(* Logix 5000 AddOnInstructionDefinition export MTRQ_Yaskawa; software revision 17.00 *)

TYPE Yaskawa_EIP_Servo :   // Yaskawa SigmaLogic Axis Structure v2.4.0
STRUCT
   O : Yaskawa_OUT_to_Servo;
   I : Yaskawa_IN_from_Servo;
   AOI_SB : Yaskawa_AOI_Status_Bits;
END_STRUCT
END_TYPE

TYPE Yaskawa_OUT_to_Servo :   // Structure of data sent out to the Yaskawa SigmaLogic controller v2.4.0
STRUCT
   b00_ServoOn : BOOL;   // Servo On
   b01_Stop : BOOL;   // Stops All Current Motion in Progress
   b02_Home : BOOL;   // Start Homing Process
   b03_MoveStart1 : BOOL;   // Start Current Motion
   b06_SuperImpose : BOOL;
   b07_ServoAlarmReset : BOOL;   // Servo Alarm Reset
   b08_ControllerAlarmReset : BOOL;   // SigmaLogic Alarm Reset
   b09_MoveStart2 : BOOL;   // Start Second Motion (Blended Move)
   b10_MoveAbort : BOOL;   // Abort Current Move
   b11_MovePause : BOOL;   // Pause Current Move
   b12_SeqPause : BOOL;   // Indexing Sequence Pause
   b13_SeqResume : BOOL;   // Indexing Sequence Resume
   b14_SeqCancel : BOOL;   // Indexing Sequence Cancel
   b15_AbsEncoderReset : BOOL;   // Absolute Encoder Reset
   b16_SeqStart : BOOL;   // Start Indexing Sequence
   b17_SeqEditSpeed : BOOL;   // Enter Edit Speed
   b18_SeqEditDistance : BOOL;   // Enter Distance Edit
   b19_PLSEnable : BOOL;   // Enable PLS execution
   b20_PLSActivateOutput1 : BOOL;   // Activate PLS output1 switch logic
   b21_PLSActivateOutput2 : BOOL;   // Activate PLS output2 switch logic
   b22_PLSActivateOutput3 : BOOL;   // Activate PLS output3 switch logic
   b23_PLSActivateOutput4 : BOOL;   // Activate PLS output4 switch logic
   b24_SetClock : BOOL;   // Set the remote controller clock with data provided by the PLC
   RebootController : BOOL;
   UseExternalEncoder : BOOL;   // Use External Encoder when executing MAHSP_Yaskawa
   b32_HeatbeatAnswer : BOOL;   // Heartbeat Answer
   BrakeBypassRequest : BOOL;
   SetFwdTorqueLimit : BOOL;
   SetRevTorqueLimit : BOOL;
   TorqueLimit : DINT;
   TorqueRamp : DINT;
   HomeMethod : INT;
   HomeSpeed : DINT;
   HomeAccDec : DINT;   // Home Move Acceleration/Deceleration Rate
   HomeBackOffDistance : DINT;
   HomeCreepSpeed : DINT;
   HomeCreepDistanceLimit : DINT;
   HomeCreepTimeLimit : DINT;
   HomeOffsetDistance : DINT;
   HomeOffsetSpeed : DINT;
   HomePostion : DINT;
   HomeTorque : DINT;
   HomeInputNo : DINT;
   HomeApproachTimeLimit : DINT;
   HomeApproachDistLimit : DINT;
   HomeDirection : INT;
   HomeSwitchMode : INT;
   MoveType : INT;
   MoveDirection : INT;
   MoveAccel1 : DINT;
   MoveAccel2 : DINT;
   MoveDecel1 : DINT;
   MoveDecel2 : DINT;
   MoveSpeed1 : DINT;
   MoveSpeed2 : DINT;
   MoveDistance1 : DINT;
   MoveDistance2 : DINT;
   MovePosition1 : DINT;
   MovePosition2 : DINT;
   RegistrationDistance : DINT;
   GearNumerator : DINT;
   GearDenominator : DINT;
   SuperImposeDistance : DINT;
   Resolution : INT;
   RegistrationDirection : INT;
   TuningLevel : INT;
   SequenceStep : INT;   // Staring Sequence Step Number
   SequenceEditStep : INT;   // Sequence Step Number to Edit
   FlagCommandBits1 : DINT;   // Flag Commands. 1..64 are General Flags, Bits 0..31 correspond to Flag 1..32
   FlagCommandBits2 : DINT;   // Flag Commands cont. 1..64 are General Flags, Bits 0..31 correspond to Flag 33..64
   DigitalOutCommandBits : DINT;   // Digital Output commands. Bits 0-7 correspond to CN13 Digital Outputs 0-7, used as Flag 73-80. Bits 8-10 correspond to CN1 Digital Outputs 0-2 used as Flag 88-90"
   SequenceEditSpeed : DINT;
   SequenceEditDistance : DINT;
   FeedRateOverride : INT;
   HSI_Enable : BOOL;
   HSI_MoveMode : BOOL;   // 0=Relative; 1=Moves per Cycle
   HSI_CalcMethod : BOOL;   // 0=Accel/Decel; 1=Time
   HSI_MoveDirection : BOOL;   // 0 = Negative; 1 = Positive
   HSI_TriggerFlag : INT;
   HSI_MovingFlag : INT;
   HSI_DwellingFlag : INT;
   HSI_DoneFlag : INT;
   HSI_MoveType : INT;   // 0=Single; 1=Repeat; 2=Repeat "x" times
   HSI_RepeatNumber : INT;
   HSI_Distance : DINT;
   HSI_Speed : DINT;
   HSI_Accel : DINT;
   HSI_MoveTime : DINT;
   HSI_DwellTime : DINT;
   PLS_OutputFlag1 : INT;
   PLS_OutputFlag2 : INT;
   PLS_OutputFlag3 : INT;
   PLS_OutputFlag4 : INT;
   PLS_OnPosition1 : DINT;
   PLS_OffPosition1 : DINT;
   PLS_OnPosition2 : DINT;
   PLS_OffPosition2 : DINT;
   PLS_OnPosition3 : DINT;
   PLS_OffPosition3 : DINT;
   PLS_OnPosition4 : DINT;
   PLS_OffPosition4 : DINT;
   PLS_OnCompensation1 : INT;
   PLS_OffCompensation1 : INT;
   PLS_OnCompensation2 : INT;
   PLS_OffCompensation2 : INT;
   PLS_OnCompensation3 : INT;
   PLS_OffCompensation3 : INT;
   PLS_OnCompensation4 : INT;
   PLS_OffCompensation4 : INT;
   RTC_Year : INT;
   RTC_Month : INT;
   RTC_Day : INT;
   RTC_Hour : INT;
   RTC_Min : INT;
   RTC_Sec : INT;
   StopDecel : DINT;
   AnalogOutput : INT;   // CN13, AO_01 [mV]
END_STRUCT
END_TYPE

TYPE Yaskawa_AOI_Status_Bits :   // Internal bits used to interlock Yaskawa AOI execution. v2.4.0
STRUCT
   MAM : BOOL;   // Move AOI Active
   MAJ : BOOL;   // Jog AOI Active
   MAB : BOOL;   // Blending AOI Active
   MAG : BOOL;   // Gearing AOI Active
   MAHSP : BOOL;   // Home SetPoint AOI Active
   MAH : BOOL;   // Homing AOI Active
   MSQE : BOOL;   // Sequence Edit AOI Active
   MSQR : BOOL;   // Sequence Run AOI Active
   MHSI : BOOL;   // High Speed Index AOI Active
   MSO : BOOL;   // Servo On
   MSF : BOOL;   // Servo Off
   MAFR : BOOL;   // Fault Reset
   MAS : BOOL;   // Servo Abort
   MTRQ : BOOL;   // Torque Mode Active
   MPLS : BOOL;   // PLS Active
   MCLK : BOOL;   // SetClock Active
   MSTL : BOOL;   // Set Torque Limit Active
   AOI_Permissive : BOOL;   // Permissive to Execute an AOI
END_STRUCT
END_TYPE

TYPE Yaskawa_IN_from_Servo :   // Structure of data coming from the Yaskawa SigmaLogic controller. v2.4.0
STRUCT
   AlarmText : STRING;   // ServoPack Alarm Code plus Text Description
   b00_Heartbeat : BOOL;
   b01_Alarm : BOOL;   // ServoPack Alarm
   b02_Warning : BOOL;   // ServoPack Warning
   b03_Ready : BOOL;   // ServoPack Ready
   b04_Enabled : BOOL;   // ServoPack Enabled ("Servo On")
   b05_StopComplete : BOOL;
   b06_HomeComplete : BOOL;
   b07_HomeBusy : BOOL;
   b08_HomeActive : BOOL;
   b09_HomeAborted : BOOL;
   b10_HomeError : BOOL;
   b11_MoveAbsComplete : BOOL;
   b12_MoveAbsBusy : BOOL;
   b13_MoveAbsActive : BOOL;
   b14_MoveAbsAborted : BOOL;
   b15_MoveAbsError : BOOL;
   b16_MoveRelComplete : BOOL;
   b17_MoveRelBusy : BOOL;
   b18_MoveRelActive : BOOL;
   b19_MoveRelAborted : BOOL;
   b20_MoveRelError : BOOL;
   b21_JogAtSpeed : BOOL;
   b22_JogBusy : BOOL;
   b23_JogActive : BOOL;
   b24_JogAborted : BOOL;
   b25_JogError : BOOL;
   b26_GearInSync : BOOL;
   b27_GearBusy : BOOL;
   b28_GearActive : BOOL;
   b29_GearAborted : BOOL;
   b30_GearError : BOOL;
   b32_MoveSuperComplete : BOOL;
   b33_MoveSuperBusy : BOOL;
   b34_MoveSuperActive : BOOL;
   b35_MoveSuperAborted : BOOL;
   b36_MoveSuperError : BOOL;
   b37_PowerCycleRequired : BOOL;
   b38_MoveBlend1Complete : BOOL;
   b39_MoveBlend1Busy : BOOL;
   b40_MoveBlend1Active : BOOL;
   b41_MoveBlend1Abort : BOOL;
   b42_MoveBlend1Error : BOOL;
   b43_MoveBlend2Complete : BOOL;
   b44_MoveBlend2Busy : BOOL;
   b45_MoveBlend2Active : BOOL;
   b46_MoveBlend2Abort : BOOL;
   b47_MoveBlend2Error : BOOL;
   b48_RegComplete : BOOL;
   b49_RegBusy : BOOL;
   b50_RegActive : BOOL;
   b51_RegAborted : BOOL;
   b52_RegError : BOOL;
   b53_ResetAbsEncoderActive : BOOL;
   b54_ResetAbsEncoderBusy : BOOL;
   b55_ResetAbsEncoderDone : BOOL;
   b56_ResetAbsEncoderError : BOOL;
   b57_SeqRunning : BOOL;
   b58_RegSensorNotReached : BOOL;
   b59_SeqEditError : BOOL;
   b60_SeqEditDone : BOOL;
   b61_TorqueAtTorque : BOOL;
   b62_TorqueBusy : BOOL;
   b63_TorqueActive : BOOL;
   b64_TorqueAborted : BOOL;
   b65_TorqueError : BOOL;
   b66_ControllerAlarm : BOOL;
   b67_ApplicationError : BOOL;
   b68_AxisAtStandStill : BOOL;
   b69_TestModeActive : BOOL;
   b70_ServoParamsOK : BOOL;
   b71_SetFwdTorqueLimitDone : BOOL;
   b72_SetRevTorqueLimitDone : BOOL;
   Position : DINT;
   Speed : DINT;
   Torque : DINT;
   HomeErrorID : INT;
   MoveAbsErrorID : INT;
   MoveRelErrorID : INT;
   JogErrorID : INT;
   GearErrorID : INT;
   MoveSuperErrorID : INT;
   ServoAlarmID : INT;
   ServoWarningID : INT;
   ControllerAlarmID : DINT;
   AxisGenAlarmID : DINT;
   MoveBlend1ErrorID : INT;
   MoveBlend2ErrorID : INT;
   ResetAbsEncoderErrorID : INT;
   FunctionBlockErrorID : INT;
   TorqueErrorID : INT;
   RegErrorID : INT;
   SeqCurrentStep : INT;
   FlagStatusBit1 : DINT;   // Flag Status. 1..64 are General Flags, Bits 0..31 correspond to Flag 1..32
   FlagStatusBit2 : DINT;   // Flag Status cont. 1..64 are General Flags, Bits 0..31 correspond to Flag 33..64
   IOStatusBits : DINT;   // Digital IO Status. Bits 0-7, CN13 Inputs 0-7, Used as Flag 65-72. Bits 8-15, CN13 Outputs 0-7, Used as Flag 73-80. Bits 16-22, CN1 Inputs 0-6, Used as Flag 81-87. Bits 23-25, CN1 Outputs 0-4, Used as Flag 88-92.
   HSI_Moving : BOOL;
   HSI_Dwelling : BOOL;
   HSI_Done : BOOL;
   HSI_Busy : BOOL;
   HSI_Error : BOOL;
   HSI_ErrorCode : INT;
   PLS_Running : BOOL;
   PLS_SwitchStatus1 : BOOL;
   PLS_SwitchStatus2 : BOOL;
   PLS_SwitchStatus3 : BOOL;
   PLS_SwitchStatus4 : BOOL;
   PLS_Busy : BOOL;
   PLS_Error : BOOL;
   PLS_ErrorCode : INT;
   SetClock_Done : BOOL;
   SetClock_Busy : BOOL;
   SetClock_Error : BOOL;
   SetClock_ErrorID : INT;
   SoftwareVersion : DINT;
   FirmwareVersion : DINT;
   CommandedPos : DINT;
   CommandedPosNonCyc : DINT;
   CommandedSpeed : DINT;
   Clock_Year : INT;
   Clock_Month : INT;
   Clock_Day : INT;
   Clock_Hour : INT;
   Clock_Minute : INT;
   Clock_Second : INT;
   AnalogInput : REAL;   // CN13, AI_01 [v]
   BrakeBypassActive : BOOL;
   ForwardTorqueLimit : DINT;
   ReverseTorqueLimit : DINT;
END_STRUCT
END_TYPE

ADD_ON_INSTRUCTION MTRQ_Yaskawa   (* revision 2.4 0, vendor Yaskawa America, Inc., ExecuteEnableInFalse *)
// Motion Axis Torque Control
// Revision note:
// 2.4.0: No functional change
// 2.3.1: Moved unlatch of AOI_ON_LOCAL to bottom of EnableInFalse routine so that outputs will be on for at least 1 scan if one-shot on EN is used.
// 2.3.0: No functional change
// 2.0.0: Improved output operation and error code reporting. Improved interlocking with embedded code.
// 1.2.0: Set the IP output to non-latch so that it can show correct status if torque command is changed.
// 1.1.0: Initial Release 9/10/2014
// Help:
// This AOI moves a servo axis indefinitely at a commanded maximum torque with an overall speed limit. The polarity of the torque determines the direction of motion. The motor speed will vary depending on the amount of resistance to motion present in the system. When the maximum torque value is reached, the IP output will signal 'In-Torque'.
VAR_IN_OUT
   Axis : Yaskawa_EIP_Servo; {required}
END_VAR
VAR_INPUT
   Torque_Limit : REAL := 50.0; {required}   // Torque Limit [%] during motion. Positive value is forward direction, Negative value is reverse direction.
   Torque_Ramp : REAL := 100.0; {required}   // Torque Ramp Rate [%/sec]
   Speed_Limit : REAL; {required}   // Maximum Absolute Speed to move the axis in [unit/s]
   Accel_Rate : REAL; {required}   // Acceleration rate of the axis in [unit/s/s]
   Decel_Rate : REAL; {required}   // Deceleration rate of the axis in [unit/s/s]
END_VAR
VAR_OUTPUT
   EN : BOOL; {visible}   // The AOI is Active
   IP : BOOL; {visible}   // The axis is holding "At Torque"
   ER : BOOL; {visible}   // An error has occurred with the Torque Control Motion
   FLT_RDY : BOOL; {visible}   // The Servo is Not Ready
   FLT_BSY : BOOL; {visible}   // There is another AOI Active for this Axis
   ErrorCode : INT; {visible}   // Torque Control ErrorID returned from the SigmaLogic axis
END_VAR
VAR
   AOI_ON_LOCAL : BOOL;
   Move_TORQUE : BOOL;
   ScaleFactor : DINT;
   stopping : BOOL;
   Finished : BOOL;   // Function is Finished
END_VAR

ROUTINE EnableInFalse   (* ladder *)
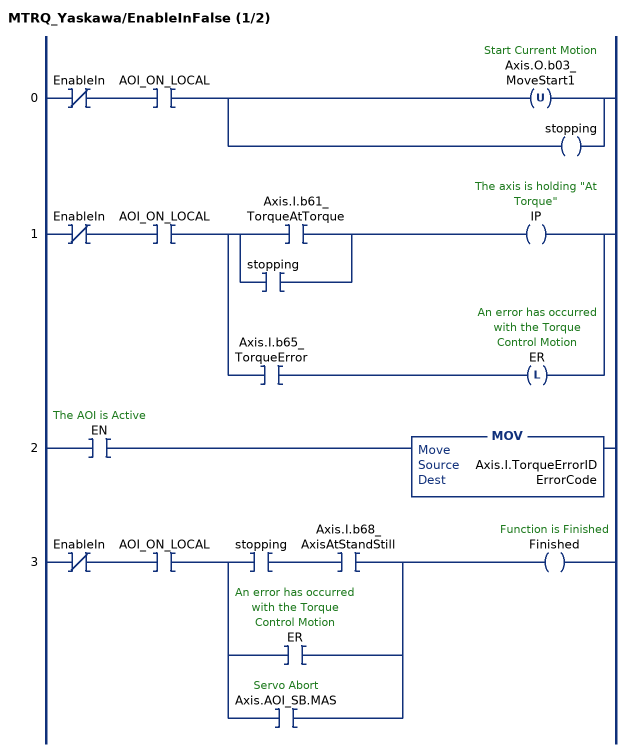
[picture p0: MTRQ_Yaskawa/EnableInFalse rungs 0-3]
   0: XIO(EnableIn)XIC(AOI_ON_LOCAL)[OTU(Axis.O.b03_MoveStart1) ,OTE(stopping) ];
   1: XIO(EnableIn)XIC(AOI_ON_LOCAL)[[XIC(Axis.I.b61_TorqueAtTorque) ,XIC(stopping) ] OTE(IP) ,XIC(Axis.I.b65_TorqueError) OTL(ER) ];
   2: XIC(EN)MOV(Axis.I.TorqueErrorID,ErrorCode);
   3: XIO(EnableIn)XIC(AOI_ON_LOCAL)[XIC(stopping) XIC(Axis.I.b68_AxisAtStandStill) ,XIC(ER) ,XIC(Axis.AOI_SB.MAS) ]OTE(Finished);
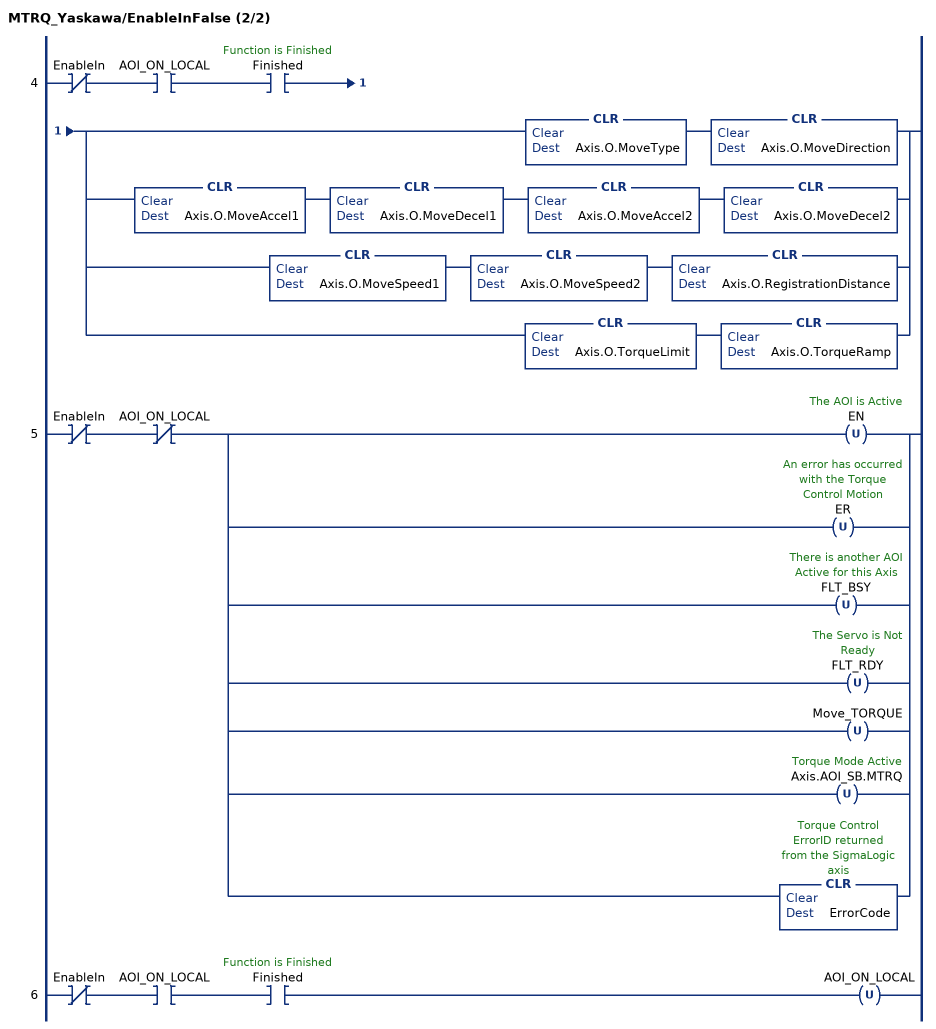
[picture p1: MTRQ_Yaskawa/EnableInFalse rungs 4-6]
   4: XIO(EnableIn)XIC(AOI_ON_LOCAL)XIC(Finished)[CLR(Axis.O.MoveType) CLR(Axis.O.MoveDirection) ,CLR(Axis.O.MoveAccel1) CLR(Axis.O.MoveDecel1) CLR(Axis.O.MoveAccel2) CLR(Axis.O.MoveDecel2) ,CLR(Axis.O.MoveSpeed1) CLR(Axis.O.MoveSpeed2) CLR(Axis.O.RegistrationDistance) ,CLR(Axis.O.TorqueLimit) CLR(Axis.O.TorqueRamp) ];
   5: XIO(EnableIn)XIO(AOI_ON_LOCAL)[OTU(EN) ,OTU(ER) ,OTU(FLT_BSY) ,OTU(FLT_RDY) ,OTU(Move_TORQUE) ,OTU(Axis.AOI_SB.MTRQ) ,CLR(ErrorCode) ];
   6: XIO(EnableIn)XIC(AOI_ON_LOCAL)XIC(Finished)OTU(AOI_ON_LOCAL);
END_ROUTINE

ROUTINE Logic   (* ladder *)
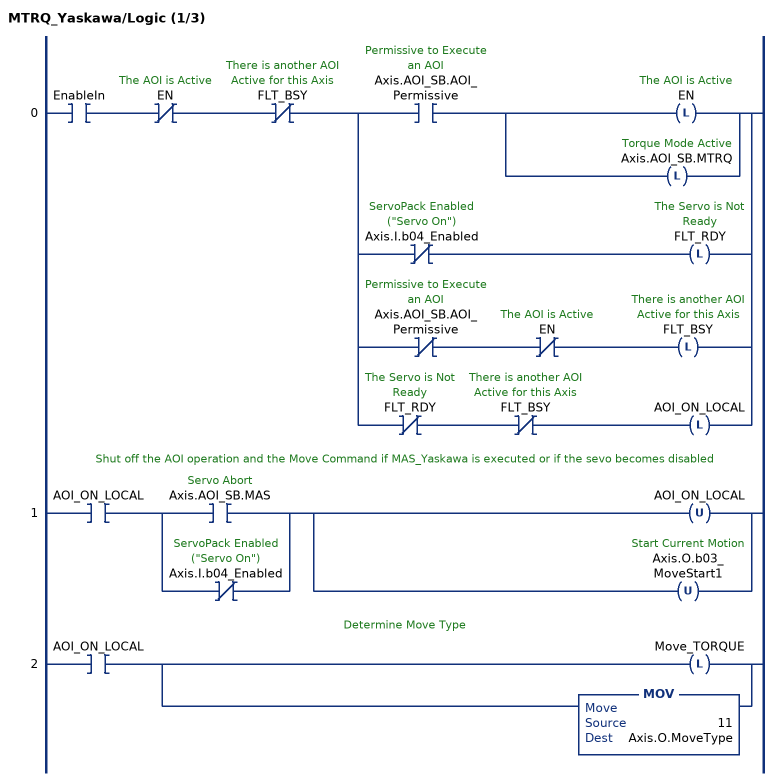
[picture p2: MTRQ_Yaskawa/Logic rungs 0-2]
   0: XIC(EnableIn)XIO(EN)XIO(FLT_BSY)[XIC(Axis.AOI_SB.AOI_Permissive) [OTL(EN) ,OTL(Axis.AOI_SB.MTRQ) ] ,XIO(Axis.I.b04_Enabled) OTL(FLT_RDY) ,XIO(Axis.AOI_SB.AOI_Permissive) XIO(EN) OTL(FLT_BSY) ,XIO(FLT_RDY) XIO(FLT_BSY) OTL(AOI_ON_LOCAL) ];
   // Shut off the AOI operation and the Move Command if MAS_Yaskawa is executed or if the sevo becomes disabled
   1: XIC(AOI_ON_LOCAL)[XIC(Axis.AOI_SB.MAS) ,XIO(Axis.I.b04_Enabled) ][OTU(AOI_ON_LOCAL) ,OTU(Axis.O.b03_MoveStart1) ];
   // Determine Move Type
   2: XIC(AOI_ON_LOCAL)[OTL(Move_TORQUE) ,MOV(11,Axis.O.MoveType) ];
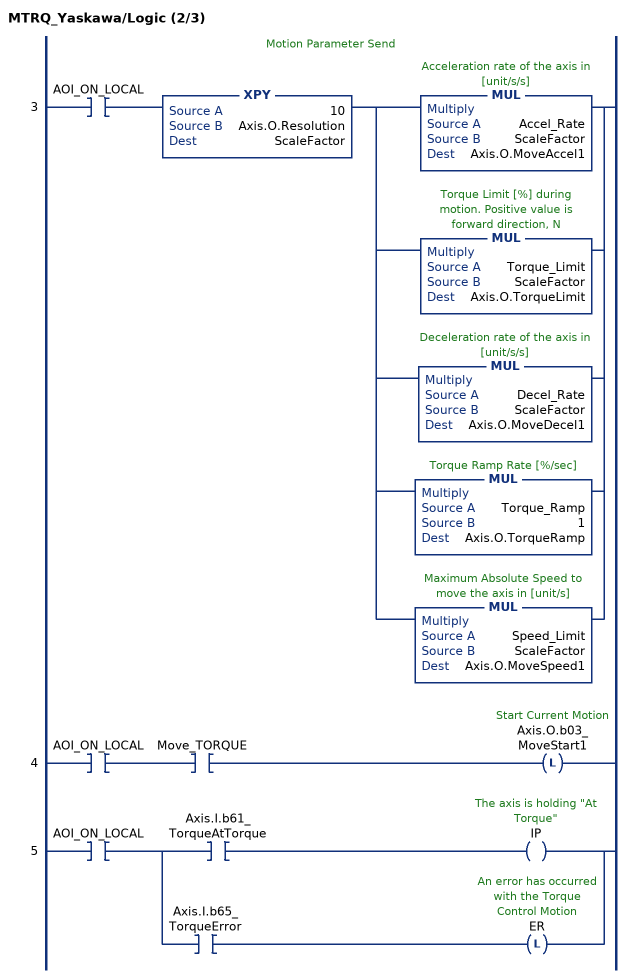
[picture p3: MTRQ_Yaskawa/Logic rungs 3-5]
   // Motion Parameter Send
   3: XIC(AOI_ON_LOCAL)XPY(10,Axis.O.Resolution,ScaleFactor)[MUL(Accel_Rate,ScaleFactor,Axis.O.MoveAccel1) ,MUL(Torque_Limit,ScaleFactor,Axis.O.TorqueLimit) ,MUL(Decel_Rate,ScaleFactor,Axis.O.MoveDecel1) ,MUL(Torque_Ramp,1,Axis.O.TorqueRamp) ,MUL(Speed_Limit,ScaleFactor,Axis.O.MoveSpeed1) ];
   4: XIC(AOI_ON_LOCAL)XIC(Move_TORQUE)OTL(Axis.O.b03_MoveStart1);
   5: XIC(AOI_ON_LOCAL)[XIC(Axis.I.b61_TorqueAtTorque) OTE(IP) ,XIC(Axis.I.b65_TorqueError) OTL(ER) ];
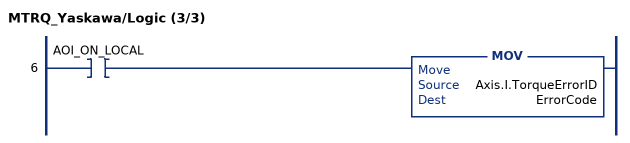
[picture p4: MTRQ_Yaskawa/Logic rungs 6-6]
   6: XIC(AOI_ON_LOCAL)MOV(Axis.I.TorqueErrorID,ErrorCode);
END_ROUTINE
END_ADD_ON_INSTRUCTION
